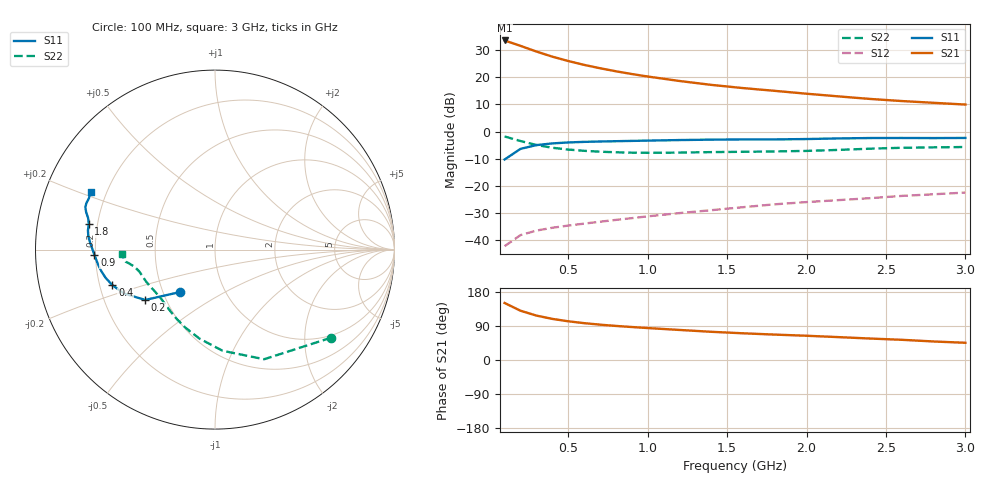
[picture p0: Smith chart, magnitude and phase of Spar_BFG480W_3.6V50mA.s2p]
! Filename: 3_650BFG480.001
! Title: BFG480W
! Bias: Vce=3.6V; Ic=50mA
! Company: NXP Semiconductors NL
! User: Quality&Reliability T&D
! Measure time: 10 Nov 1999 / 11:59:58
#  MHz  S  MA  R 50
! Freq  S11  S21  S12  S22  :
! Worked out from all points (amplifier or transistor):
!   20 points, 100 MHz to 3 GHz, reference 50 ohm
!   highest |S21| = 33.6 dB at 100 MHz (marker M1)
!   |S21| within 3 dB of that: start of sweep to 247.9 MHz
!   unconditionally stable (mu >= 1): 955.4 MHz to end of sweep
!   at 400 MHz: K = 0.64, MSG = 31.6 dB, |S12| = -35.5 dB
!   at 1.2 GHz: K = 1.05, MAG = 23.0 dB, |S12| = -30.1 dB
!   at 3 GHz: K = 1.06, MAG = 14.7 dB, |S12| = -22.5 dB
!   S11 on the Smith chart (normalised r, x): 100 MHz: 0.61, -0.32; 200 MHz: 0.38, -0.28; 400 MHz: 0.25, -0.16; 900 MHz: 0.20, -0.02; 1.8 GHz: 0.17, +0.10; 3 GHz: 0.14, +0.22
100  0.305 -129.3  48.12 150.4  0.007661 67.0  0.8119 -37.2
200  0.4795 -144.2  38.24 130.1  0.01226 56.9  0.6694 -65.8
300  0.5623 -154.2  30.04 117.2  0.01486 53.2  0.5653 -85.7
400  0.6047 -160.8  24.19 108.5  0.01674 52.6  0.503 -100.0
500  0.6298 -165.6  20.09 102.2  0.01837 53.7  0.4654 -110.7
600  0.6453 -169.4  17.05 97.2  0.01996 55.4  0.4416 -118.8
700  0.6558 -172.4  14.78 93.3  0.02166 57.6  0.4255 -125.2
800  0.6641 -175.1  12.99 89.9  0.0234 59.5  0.4147 -130.6
900  0.6725 -177.5  11.55 87.0  0.0252 61.6  0.4083 -135.2
1000  0.6809 -179.7  10.39 84.3  0.02722 63.2  0.4057 -139.4
1200  0.6974 176.7  8.594 79.3  0.03124 66.0  0.4092 -146.3
1400  0.7097 174.0  7.285 74.4  0.03534 68.0  0.4176 -151.5
1600  0.716 171.4  6.354 70.5  0.04017 69.7  0.4234 -155.4
1800  0.7171 168.6  5.65 67.0  0.0454 71.0  0.4298 -159.4
2000  0.7279 166.1  5.002 64.0  0.04992 72.3  0.4395 -164.0
2200  0.7477 163.8  4.465 60.4  0.05423 72.7  0.4586 -168.0
2400  0.76 161.9  4.005 56.7  0.05896 72.6  0.4831 -170.7
2600  0.7621 160.2  3.661 53.3  0.06492 72.4  0.5021 -172.3
2800  0.7583 157.9  3.396 48.9  0.06957 71.4  0.5112 -174.3
3000  0.7634 155.2  3.153 45.4  0.07485 70.8  0.5187 -177.4
